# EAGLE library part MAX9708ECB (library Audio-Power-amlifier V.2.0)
The MAX9708 mono/stereo, Class D audio power amplifier delivers up to 2 x 21W into an 8Ω stereo mode and 1 x 42W into a 4Ω load in mono mode while offering up to 87% efficiency. The MAX9708 provides Class AB amplifier performance with the benefits of Class D efficiency, eliminating the need for a bulky heatsink and conserving power. The MAX9708 operates from a single +10V to +18V supply, driving the load in a BTL configuration. The MAX9708
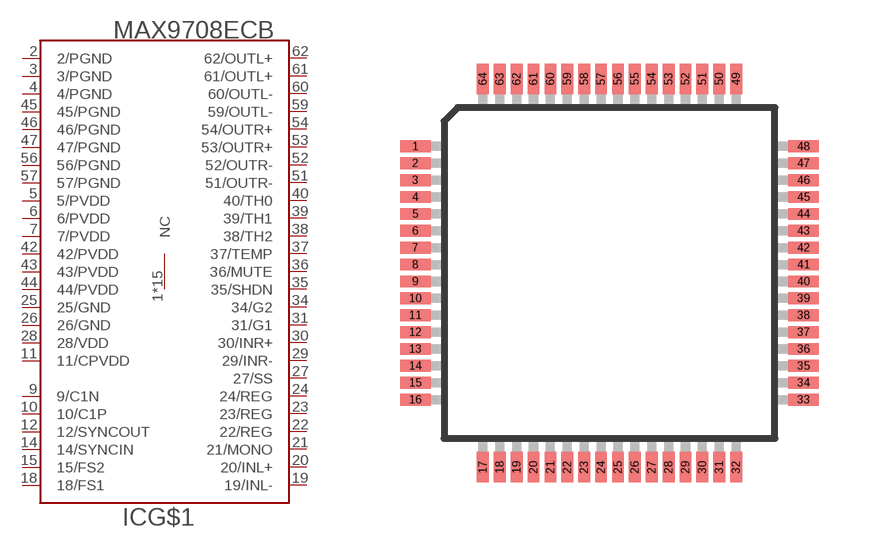
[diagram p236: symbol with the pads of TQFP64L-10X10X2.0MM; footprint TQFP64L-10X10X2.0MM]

Designator prefix IC; gates G$1=MAX9708ECB G$2=NC

## MAX9708ECBMAX9708ECB  [TQFP64L-10X10X2.0MM]
1  G$2:NC  nc
2  G$1:2/PGND  pwr
3  G$1:3/PGND  pwr
4  G$1:4/PGND  pwr
5  G$1:5/PVDD  pwr
6  G$1:6/PVDD  pwr
7  G$1:7/PVDD  pwr
8  G$2:NC  nc
9  G$1:9/C1N
10  G$1:10/C1P
11  G$1:11/CPVDD  pwr
12  G$1:12/SYNCOUT  out
13  G$2:NC  nc
14  G$1:14/SYNCIN  in
15  G$1:15/FS2
16  G$2:NC  nc
17  G$2:NC  nc
18  G$1:18/FS1
19  G$1:19/INL-  in
20  G$1:20/INL+  in
21  G$1:21/MONO  in
22  G$1:22/REG  out
23  G$1:23/REG  out
24  G$1:24/REG  out
25  G$1:25/GND  pwr
26  G$1:26/GND  pwr
27  G$1:27/SS
28  G$1:28/VDD  pwr
29  G$1:29/INR-  in
30  G$1:30/INR+  in
31  G$1:31/G1  in
32  G$2:NC  nc
33  G$2:NC  nc
34  G$1:34/G2  in
35  G$1:35/SHDN  in
36  G$1:36/MUTE  in
37  G$1:37/TEMP  out
38  G$1:38/TH2  in
39  G$1:39/TH1  in
40  G$1:40/TH0  in
41  G$2:NC  nc
42  G$1:42/PVDD  pwr
43  G$1:43/PVDD  pwr
44  G$1:44/PVDD  pwr
45  G$1:45/PGND  pwr
46  G$1:46/PGND  pwr
47  G$1:47/PGND  pwr
48  G$2:NC  nc
49  G$2:NC  nc
50  G$2:NC  nc
51  G$1:51/OUTR-  out
52  G$1:52/OUTR-  out
53  G$1:53/OUTR+  out
54  G$1:54/OUTR+  out
55  G$2:NC  nc
56  G$1:56/PGND  pwr
57  G$1:57/PGND  pwr
58  G$2:NC  nc
59  G$1:59/OUTL-  out
60  G$1:60/OUTL-  out
61  G$1:61/OUTL+  out
62  G$1:62/OUTL+  out
63  G$2:NC  nc
64  G$2:NC  nc

## Footprint TQFP64L-10X10X2.0MM (pad centres in mm)
TQFP 64L-10X10X1,4 MM www.maxim-ic.com/packages
smd 0.9 x 0.35: 1 -5.75,3.75; 2 -5.75,3.25; 3 -5.75,2.75; 4 -5.75,2.25; 5 -5.75,1.75; 6 -5.75,1.25; 7 -5.75,0.75; 8 -5.75,0.25; 9 -5.75,-0.25; 10 -5.75,-0.75; 11 -5.75,-1.25; 12 -5.75,-1.75; 13 -5.75,-2.25; 14 -5.75,-2.75; 15 -5.75,-3.25; 16 -5.75,-3.75; 33 5.75,-3.75; 34 5.75,-3.25; 35 5.75,-2.75; 36 5.75,-2.25; 37 5.75,-1.75; 38 5.75,-1.25; 39 5.75,-0.75; 40 5.75,-0.25; 41 5.75,0.25; 42 5.75,0.75; 43 5.75,1.25; 44 5.75,1.75; 45 5.75,2.25; 46 5.75,2.75; 47 5.75,3.25; 48 5.75,3.75
smd 0.35 x 0.9: 17 -3.75,-5.75; 18 -3.25,-5.75; 19 -2.75,-5.75; 20 -2.25,-5.75; 21 -1.75,-5.75; 22 -1.25,-5.75; 23 -0.75,-5.75; 24 -0.25,-5.75; 25 0.25,-5.75; 26 0.75,-5.75; 27 1.25,-5.75; 28 1.75,-5.75; 29 2.25,-5.75; 30 2.75,-5.75; 31 3.25,-5.75; 32 3.75,-5.75; 49 3.75,5.75; 50 3.25,5.75; 51 2.75,5.75; 52 2.25,5.75; 53 1.75,5.75; 54 1.25,5.75; 55 0.75,5.75; 56 0.25,5.75; 57 -0.25,5.75; 58 -0.75,5.75; 59 -1.25,5.75; 60 -1.75,5.75; 61 -2.25,5.75; 62 -2.75,5.75; 63 -3.25,5.75; 64 -3.75,5.75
